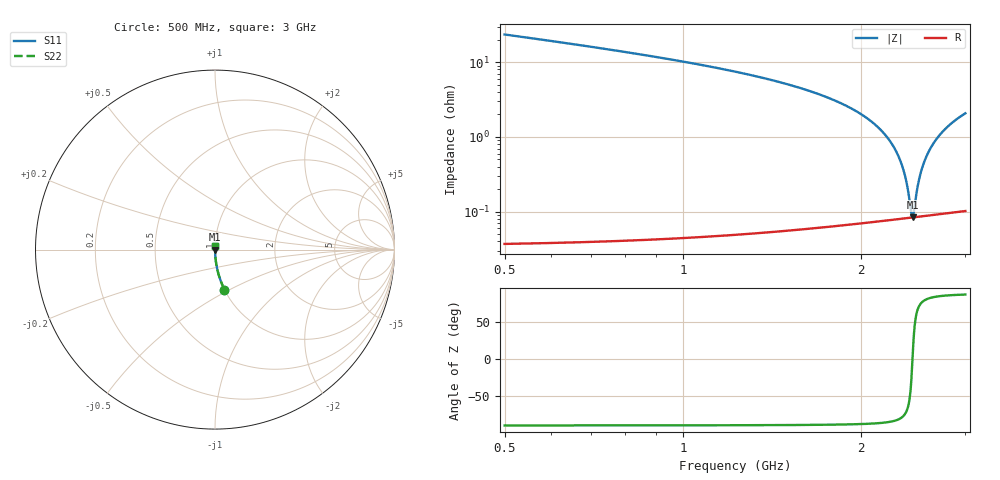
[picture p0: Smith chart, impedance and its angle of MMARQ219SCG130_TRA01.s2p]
! MMARQ219SCG130_TRA01  S-PARAMETER MODEL  ( General Type )
! Model Generated by TAIYO YUDEN Corporation (http://www.ty-top.com)
! Version 1.0
! TAIYO YUDEN Control No. 180601
! Copyright(c) 2018 TAIYO YUDEN CO.,LTD. All Rights Reserved.
! Product Description (link to TY-COMPAS)
! https://ds.yuden.co.jp/TYCOMPAS/or/detail?pn=MMARQ219SCG130JTRA01&u=M
! Products Name : Multilayer Ceramic Capacitors
! Characteristics :
!  Capacitance : 13 pF , Rated Voltage : 250V , TCC : CG / C0G
!  Case Size : 2.0 x 1.25 / 0.079 x 0.049 [mm/inch] , Thickness : 0.85 / 0.033 [mm/inch]
!  (Conditions: Temperature = 25 degC , DC Bias Current/Voltage = 0A / 0V)
! External Node Assignments :
!  1  o---| |---o  2
! GND o---------o GND
! Frequency Range : 500MHz  -  3000MHz  [ 401 STEP ]
# MHz S RI R 50
! Freq[MHz].  S11 Real  S11 Imag  S21 Real  S21 Imag  S12 Real  S12 Imag  S22 Real  S22 Imag
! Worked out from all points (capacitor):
!   401 points, 500 MHz to 3 GHz, reference 50 ohm
!   read as one part in series: C = 13 pF near 512.5 MHz
!   lowest |Z| = 83.9 mohm at 2.444 GHz (marker M1)
!   series resonance near 2.442 GHz, so ESL is about 330 pH
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500  0.0526 -0.2224  0.9474 0.2224  0.9474 0.2224  0.0526 -0.2224
918.75  0.0133 -0.1129  0.9867 0.1129  0.9867 0.1129  0.0133 -0.1129
1337.5  0.0046 -0.0638  0.9954 0.0638  0.9954 0.0638  0.0046 -0.0638
1750  0.00178 -0.0339  0.9982 0.0339  0.9982 0.0339  0.00178 -0.0339
1993.75  0.00111 -0.0204  0.9989 0.0204  0.9989 0.0204  0.00111 -0.0204
2168.75  0.00089 -0.0119  0.9991 0.0119  0.9991 0.0119  0.00089 -0.0119
2268.75  0.000835 -0.00737  0.9992 0.00737  0.9992 0.00737  0.000835 -0.00737
2337.5  0.000821 -0.00438  0.9992 0.00438  0.9992 0.00438  0.000821 -0.00438
2362.5  0.000821 -0.00332  0.9992 0.00332  0.9992 0.00332  0.000821 -0.00332
2381.25  0.000823 -0.00253  0.9992 0.00253  0.9992 0.00253  0.000823 -0.00253
2400  0.000825 -0.00175  0.9992 0.00175  0.9992 0.00175  0.000825 -0.00175
2431.25  0.000833 -0.000454  0.9992 0.000454  0.9992 0.000454  0.000833 -0.000454
2443.75  0.000836 5.83e-05  0.9992 -5.83e-05  0.9992 -5.83e-05  0.000836 5.83e-05
2456.25  0.000841 0.000568  0.9992 -0.000568  0.9992 -0.000568  0.000841 0.000568
2487.5  0.000854 0.00183  0.9991 -0.00183  0.9991 -0.00183  0.000854 0.00183
2512.5  0.000867 0.00283  0.9991 -0.00283  0.9991 -0.00283  0.000867 0.00283
2543.75  0.000886 0.00406  0.9991 -0.00406  0.9991 -0.00406  0.000886 0.00406
2587.5  0.000917 0.00577  0.9991 -0.00577  0.9991 -0.00577  0.000917 0.00577
2656.25  0.000976 0.00839  0.999 -0.00839  0.999 -0.00839  0.000976 0.00839
2750  0.00108 0.0119  0.9989 -0.0119  0.9989 -0.0119  0.00108 0.0119
2868.75  0.00124 0.0161  0.9988 -0.0161  0.9988 -0.0161  0.00124 0.0161
3000  0.00145 0.0206  0.9986 -0.0206  0.9986 -0.0206  0.00145 0.0206
